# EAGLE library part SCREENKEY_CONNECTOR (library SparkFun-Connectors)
Connector for the ScreenKey This is a tiny, locking 14-pin FPC/FFC connector that mates with the TFT ScreenKeys and their displays. These connectors require a really minimal amount of force to close, which is great for the delicate wires they’re designed for. Unfortunately, we no longer sell the ScreenKey TFT128 or the TFT128 Display, however we do still sell the connector. Here is the connector we sell at SparkFun: ScreenKey Mating Connector (PRT-09586) Datasheet (FH12-14S-0.5SH)
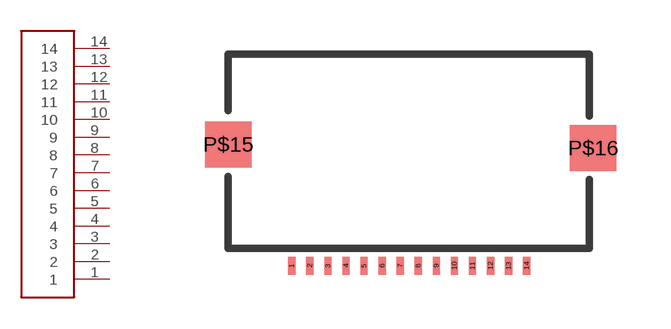
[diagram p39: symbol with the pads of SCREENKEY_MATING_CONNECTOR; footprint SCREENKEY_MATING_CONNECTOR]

Designator prefix J

## SCREENKEY_CONNECTOR (PROD_ID: CONN-09581; SF_ID: PRT-09586)  [SCREENKEY_MATING_CONNECTOR]
1  1
2  2
3  3
4  4
5  5
6  6
7  7
8  8
9  9
10  10
11  11
12  12
13  13
14  14

## Footprint SCREENKEY_MATING_CONNECTOR (pad centres in mm)
FPC/FFC Locking Connector - SMD Specifications: Pin count:14 Pin pitch: 0.5mm Datasheet referenced for footprint Example device(s): SCREENKEY_CONNECTOR
smd 0.2 x 0.5: 1 1.76,-0.36; 2 2.26,-0.36; 3 2.76,-0.36; 4 3.26,-0.36; 5 3.76,-0.36; 6 4.26,-0.36; 7 4.76,-0.36; 8 5.26,-0.36; 9 5.76,-0.36; 10 6.26,-0.36; 11 6.76,-0.36; 12 7.26,-0.36; 13 7.76,-0.36; 14 8.26,-0.36
smd 1.28 x 1.28: P$15 0,3; P$16 10.1,2.9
